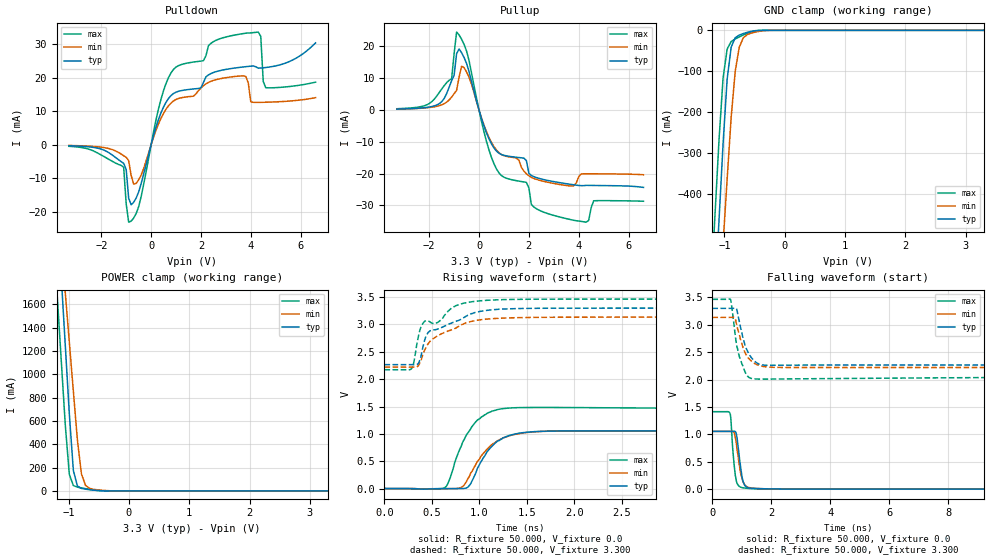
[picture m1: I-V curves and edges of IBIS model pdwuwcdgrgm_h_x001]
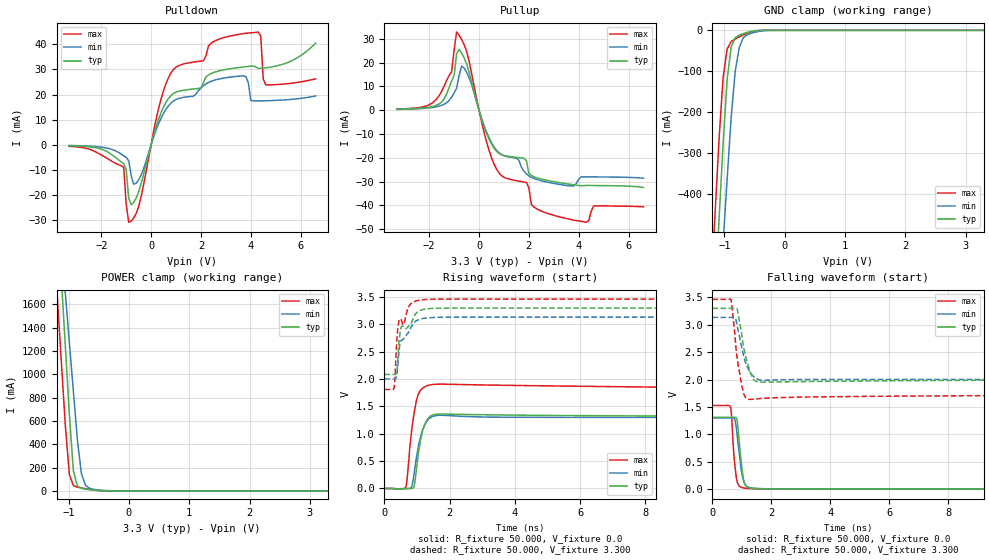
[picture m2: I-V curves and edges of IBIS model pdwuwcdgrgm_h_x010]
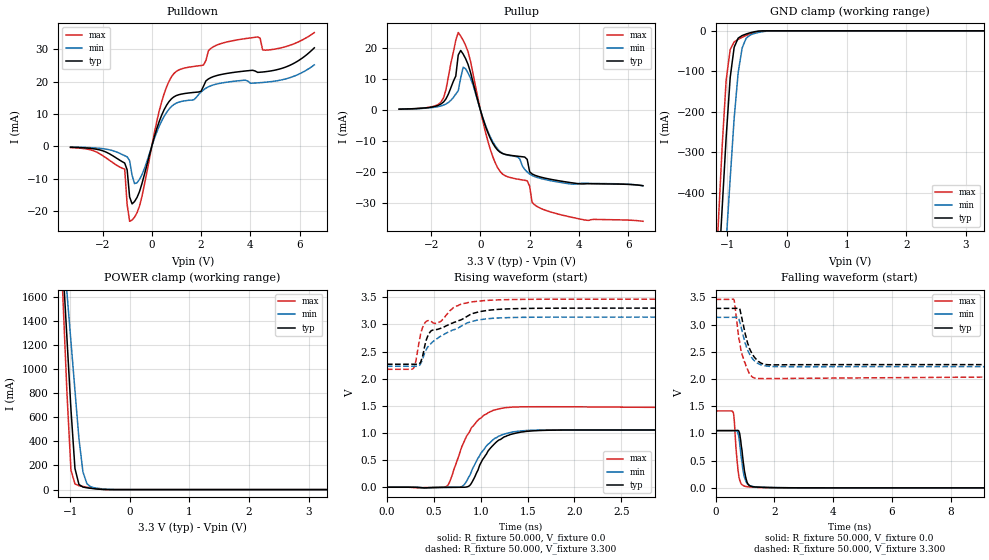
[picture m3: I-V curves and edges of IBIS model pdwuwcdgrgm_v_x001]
|   IBIS Model of Analog Devices ADSP-SC569
|   ADSP Device
[IBIS ver]   4.2
[File name]   adsc565.ibs
[File Rev]   1.0
[Date]   Fri Nov 29 10:39:13 IST 2019
[Source]   TSMC 28nm custom IO cells
[Notes]
|  GriffinUltraLite product standard
|This IBIS model is generated automatically using script /cad/local/apps/adi/ibis_gen/1.0/bin/chip_ibis_model_gen.pl
|No models exist for the following pins
|   ( Using type NC as a placeholder ):
|CLKIN_IN
|VIN0
|VIN1
|VIN2
|VIN3
|VREF_N_ADC
|VREF_P_ADC
[Disclaimer] Model intended for simulation purpose only.
[Copyright]   Property of Analog Devices Inc. Unauthorized reproduction and/or distribution is strictly prohibited.
[Component]   ADSP-SC569
[Manufacturer] Analog Devices Inc.
[Package]
|  variable   typ   min   max
R_pkg   339.97m   176.67m   530.1m
L_pkg   5.53nH   4.7nH   6.78nH
C_pkg   0.78pF   0.58pF   1.14pF
[Pin]   signal_name   model_name   R_pin   L_pin   C_pin
1	VDD_INT		POWER   NA	NA	NA
2	GND		GND   NA	NA	NA
3	VDD_INT		POWER   NA	NA	NA
4	VDD_INT		POWER   NA	NA	NA
5	CLKIN		NC   NA	NA	NA
6	XTAL		NC   NA	NA	NA
7	VDD_REF_EXT	POWER   NA	NA	NA
8	VDD_INT		POWER   NA	NA	NA
9	TEST		PDWUWCDGRGM_H			NA	NA	NA
10	CLKOUT		PDWUWCDGRGM_H			NA	NA	NA
11	VDD_REF_EXT	POWER   NA	NA	NA
12	VDD_EXT		POWER   NA	NA	NA
13	VDD_INT		POWER   NA	NA	NA
14	PA0		PDWUWCDGRGM_H			NA	NA	NA
15	PA1		PDWUWCDGRGM_H			NA	NA	NA
16	PA2		PDWUWCDGRGM_H			NA	NA	NA
17	VDD_INT		POWER   NA	NA	NA
18	PA3		PDWUWCDGRGM_H			NA	NA	NA
19	PA4		PDWUWCDGRGM_H			NA	NA	NA
20	PA5		PDWUWCDGRGM_H			NA	NA	NA
21	PA6		PDWUWCDGRGM_H			NA	NA	NA
22	VDD_INT		POWER   NA	NA	NA
23	VDD_REF_EXT	POWER   NA	NA	NA
24	VDD_EXT		POWER   NA	NA	NA
25	PA7		PDWUWCDGRGM_H			NA	NA	NA
26	PA8		PDWUWCDGRGM_H			NA	NA	NA
27	PA9		PDWUWCDGRGM_H			NA	NA	NA
28	PA10		PDWUWCDGRGM_H			NA	NA	NA
29	VDD_INT		POWER   NA	NA	NA
30	GND		GND   NA	NA	NA
31	GND		GND   NA	NA	NA
32	VDD_INT		POWER   NA	NA	NA
33	VDD_INT		POWER   NA	NA	NA
34	PA11		PDWUWCDGRGM_V			NA	NA	NA
35	PA12		PDWUWCDGRGM_V			NA	NA	NA
36	PA13		PDWUWCDGRGM_V			NA	NA	NA
37	PA14		PDWUWCDGRGM_V			NA	NA	NA
38	VDD_EXT		POWER   NA	NA	NA
39	VDD_REF_EXT	POWER   NA	NA	NA
40	PA15		PDWUWCDGRGM_V			NA	NA	NA
41	DAI0_P01	PDWUWCDGRGM_V			NA	NA	NA
42	DAI0_P02	PDWUWCDGRGM_V			NA	NA	NA
43	DAI0_P03	PDWUWCDGRGM_V			NA	NA	NA
44	VDD_INT		POWER   NA	NA	NA
45	VDD_INT		POWER   NA	NA	NA
46	DAI0_P04	PDWUWCDGRGM_V			NA	NA	NA
47	DAI0_P05	PDWUWCDGRGM_V			NA	NA	NA
48	DAI0_P06	PDWUWCDGRGM_V			NA	NA	NA
49	DAI0_P07	PDWUWCDGRGM_V			NA	NA	NA
50	VDD_EXT		POWER   NA	NA	NA
51	VDD_REF_EXT	POWER   NA	NA	NA
52	DAI0_P08	PDWUWCDGRGM_V			NA	NA	NA
53	DAI0_P09	PDWUWCDGRGM_V			NA	NA	NA
54	DAI0_P10	PDWUWCDGRGM_V			NA	NA	NA
55	DAI0_P19	PDWUWCDGRGM_V			NA	NA	NA
56	DAI0_P20	PDWUWCDGRGM_V			NA	NA	NA
57	VDD_INT		POWER   NA	NA	NA
58	GND		GND   NA	NA	NA
59	VDD_INT		POWER   NA	NA	NA
60	VDD_INT		POWER   NA	NA	NA
61	VDD_INT		POWER   NA	NA	NA
62	GND		GND   NA	NA	NA
63	DAI1_P20	PDWUWCDGRGM_H			NA	NA	NA
64	DAI1_P19	PDWUWCDGRGM_H			NA	NA	NA
65	DAI1_P10	PDWUWCDGRGM_H			NA	NA	NA
66	DAI1_P09	PDWUWCDGRGM_H			NA	NA	NA
67	VDD_REF_EXT	POWER   NA	NA	NA
68	VDD_EXT	POWER   NA	NA	NA
69	VDD_INT	POWER   NA	NA	NA
70	DAI1_P08	PDWUWCDGRGM_H			NA	NA	NA
71	DAI1_P07	PDWUWCDGRGM_H			NA	NA	NA
72	DAI1_P06	PDWUWCDGRGM_H			NA	NA	NA
73	DAI1_P05	PDWUWCDGRGM_H			NA	NA	NA
74	DAI1_P04	PDWUWCDGRGM_H			NA	NA	NA
75	DAI1_P03	PDWUWCDGRGM_H			NA	NA	NA
76	DAI1_P02	PDWUWCDGRGM_H			NA	NA	NA
77	DAI1_P01	PDWUWCDGRGM_H			NA	NA	NA
78	VDD_EXT		POWER   NA	NA	NA
79	VDD_REF_EXT	POWER   NA	NA	NA
80	VDD_INT		POWER   NA	NA	NA
81	VIN0		NC   NA	NA	NA
82	VIN1		NC   NA	NA	NA
83	VREF_P_ADC	NC   NA	NA	NA
84	VREF_N_ADC	NC   NA	NA	NA
85	VDD_A		POWER   NA	NA	NA
86	AGND		GND   NA	NA	NA
87	VDD_INT		POWER   NA	NA	NA
88	VDD_INT		POWER   NA	NA	NA
89	VDD_INT		POWER   NA	NA	NA
90	GND		GND   NA	NA	NA
91	VDD_INT		POWER   NA	NA	NA
92	GND		GND   NA	NA	NA
93	VDD_INT		POWER   NA	NA	NA
94	VDD_INT		POWER   NA	NA	NA
95	VDD_INT		POWER   NA	NA	NA
96	TDI		PDWUWCDGRGM_V			NA	NA	NA
97	TCK		PDWUWCDGRGM_V			NA	NA	NA
98	TMS		PDWUWCDGRGM_V			NA	NA	NA
99	TDO		PDWUWCDGRGM_V			NA	NA	NA
100	VDD_REF_EXT	POWER   NA	NA	NA
101	VDD_EXT		POWER   NA	NA	NA
102	FAULTb		PDWUWCDGRGM_V			NA	NA	NA
103	TRSTB		PDWUWCDGRGM_V			NA	NA	NA
104	RESETb		PDWUWCDGRGM_V			NA	NA	NA
105	BMODE0		PDWUWCDGRGM_V			NA	NA	NA
106	BMODE1		PDWUWCDGRGM_V			NA	NA	NA
107	RESOUTb		PDWUWCDGRGM_V			NA	NA	NA
108	PB0		PDWUWCDGRGM_V			NA	NA	NA
109	PB1		PDWUWCDGRGM_V			NA	NA	NA
110	VDD_INT		POWER   NA	NA	NA
111	VDD_EXT		POWER   NA	NA	NA
112	VDD_REF_EXT	POWER   NA	NA	NA
113	PB2		PDWUWCDGRGM_V			NA	NA	NA
114	PB3		PDWUWCDGRGM_V			NA	NA	NA
115	PB4		PDWUWCDGRGM_V			NA	NA	NA
116	PB5		PDWUWCDGRGM_V			NA	NA	NA
117	VDD_INT		POWER   NA	NA	NA
118	VDD_INT		POWER   NA	NA	NA
119	VDD_INT		POWER   NA	NA	NA
120	GND		GND   NA	NA	NA
|[Diff Pin] inv_pin   vdiff   tdelay_typ tdelay_min tdelay_max
[Model Selector] PDWUWCDGRGM_H
pdwuwcdgrgm_h_x001 Vbus 3.3V
pdwuwcdgrgm_h_x010 Vbus 3.3V
[Model Selector] PDWUWCDGRGM_V
pdwuwcdgrgm_v_x001 Vbus 3.3V
pdwuwcdgrgm_v_x010 Vbus 3.3V
| Models and submodels in the file (4): pdwuwcdgrgm_h_x001 (I/O), pdwuwcdgrgm_h_x010 (I/O), pdwuwcdgrgm_v_x001 (I/O), pdwuwcdgrgm_v_x010 (I/O)
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|   Model pdwuwcdgrgm_h
[Model] pdwuwcdgrgm_h_x001
Model_type I/O
Polarity   Non-Inverting
Enable   Active-Low
Vinl =  0.660V
Vinh =  2.640V
C_comp   1.489pF   1.448pF   1.508pF
C_comp_pullup   0.648pF   0.610pF   0.663pF
C_comp_pulldown   0.433pF   0.404pF   0.445pF
[Model Spec]
Vinh   2.640V   2.508V   2.772V
Vinl   0.660V   0.627V   0.693V
[Temperature Range]   25.000   0.125k   -40.000
[Voltage Range]   3.300V   3.135V   3.465V
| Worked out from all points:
|   slope of the pulldown table from 0 to 0.495 V, typ, clamps not added: 44.1 ohm
|   slope of the pullup table from 0 to 0.495 V, typ, clamps not added: 46.9 ohm
|   GND clamp passes 1 mA (typ) near -0.49 V on its own axis
|   POWER clamp passes 1 mA (typ) near -0.44 V on its own axis
|   rising waveform, R_fixture 50.000, V_fixture 0.0: 20-80 % time 232ps typ, 277ps min, 213ps max; typ from 0 V to 1.05 V
|   rising waveform, R_fixture 50.000, V_fixture 3.300: 20-80 % time 414ps typ, 371ps min, 331ps max; typ from 2.27 V to 3.3 V
|   falling waveform, R_fixture 50.000, V_fixture 0.0: 20-80 % time 151ps typ, 192ps min, 127ps max; typ from 1.05 V to 0 V
|   falling waveform, R_fixture 50.000, V_fixture 3.300: 20-80 % time 336ps typ, 361ps min, 222ps max; typ from 3.3 V to 2.27 V
[Pulldown]
|Voltage   I(typ)   I(min)   I(max)
-3.3V     -279uA     -202.5uA   -451.9uA
-1.1V     -5.541mA   -3.26mA    -6.734mA
-900mV    -15.94mA   -4.725mA   -23.11mA
-600mV    -15.91mA   -11.54mA   -20.53mA
400mV     9.624mA    7.961mA    13.71mA
1V        15.72mA    13.54mA    23.21mA
3.7V      23.25mA    20.61mA    33.22mA
4.3V      22.89mA    12.67mA    33.66mA
4.4V      22.93mA    12.68mA    32.39mA
4.5V      23mA       12.7mA     18.9mA
4.6V      23.08mA    12.71mA    17.05mA
6.6V      30.44mA    14.08mA    18.71mA
[Pullup]
|Voltage   I(typ)   I(min)   I(max)
-3.3V     304.3uA    281.9uA    413.9uA
-1.6V     1.978mA    1.36mA     5.473mA
-1.1V     9.211mA    4.075mA    9.817mA
-900mV    17.72mA    6.178mA    24.51mA
-600mV    16.54mA    13.33mA    20.64mA
600mV     -11.92mA   -11.52mA   -16.89mA
1.9V      -15.87mA   -20.02mA   -22.75mA
2.2V      -20.94mA   -21.51mA   -30.47mA
3.7V      -23.38mA   -23.88mA   -34.48mA
4.3V      -23.68mA   -20.04mA   -35.25mA
4.6V      -23.71mA   -20.04mA   -28.52mA
6.6V      -24.32mA   -20.34mA   -28.67mA
[GND_clamp]
|Voltage   I(typ)   I(min)   I(max)
-3.3V     -6.697A    -5.899A    -6.429A
-1.223V   -834.6mA   -989.4mA   -634mA
-1.156V   -647.4mA   -832.1mA   -449.2mA
-1.089V   -461.1mA   -675.2mA   -265.6mA
-1.022V   -276.3mA   -518.8mA   -115.9mA
-955mV    -119.5mA   -363.1mA   -45.68mA
-888mV    -40.94mA   -211.7mA   -27.28mA
-821mV    -18.09mA   -100.2mA   -21.05mA
-754mV    -11.69mA   -41.38mA   -15.99mA
-620mV    -4.821mA   -10.31mA   -7.225mA
-352mV    -29.83uA   -1.016mA   -30.26uA
3.3V      0A         0A         0A
[POWER_clamp]
|Voltage   I(typ)   I(min)   I(max)
-3.3V     21.13A     15.96A     19.27A
-1.189V   2.428A     2.545A     1.676A
-1.122V   1.837A     2.122A     1.121A
-1.055V   1.249A     1.699A     567.8mA
-988mV    663mA      1.276A     141.6mA
-921mV    174.9mA    855.3mA    46.28mA
-854mV    42.62mA    437.1mA    32.31mA
-787mV    21.33mA    146.3mA    25.61mA
-720mV    15.03mA    48.41mA    19.6mA
-653mV    10.52mA    22.14mA    14.03mA
-251mV    4.083uA    411.2uA    1.265uA
3.3V      0A         0A         0A
[Ramp]
| variable   typ   min   max
dV/dt_r   0.632/0.236n   0.632/0.277n   0.849/0.212n
dV/dt_f   0.621/0.334n   0.549/0.363n   0.779/0.229n
R_load = 50.000
[Rising Waveform]
R_fixture= 50.000
V_fixture= 0.0
V_fixture_min= 0.0
V_fixture_max= 0.0
|time   V(typ)   V(min)   V(max)
0s        334.6nV    124uV      235.4nV
640ps     -2.231mV   -1.827mV   21.16mV
690ps     -1.679mV   -1.21mV    184.2mV
800ps     -473uV     12.93mV    742mV
870ps     15.55mV    151.4mV    994.1mV
980ps     369.5mV    495.7mV    1.252V
1.08ns    669.5mV    715mV      1.374V
1.19ns    864.1mV    873.9mV    1.443V
1.47ns    1.024V     1.018V     1.482V
100ns     1.054V     1.054V     1.414V
[Rising Waveform]
R_fixture= 50.000
V_fixture= 3.300
V_fixture_min= 3.135
V_fixture_max= 3.465
|time   V(typ)   V(min)   V(max)
0s        2.265V     2.22V      2.173V
280ps     2.265V     2.22V      2.182V
310ps     2.265V     2.22V      2.31V
360ps     2.294V     2.253V     2.799V
410ps     2.618V     2.472V     3.031V
480ps     2.883V     2.692V     3.047V
750ps     3.056V     2.933V     3.343V
1ns       3.238V     3.083V     3.432V
1.53ns    3.295V     3.129V     3.462V
100ns     3.3V       3.135V     3.465V
[Falling Waveform]
R_fixture= 50.000
V_fixture= 0.0
V_fixture_min= 0.0
V_fixture_max= 0.0
|time   V(typ)   V(min)   V(max)
0s        1.054V     1.054V     1.414V
600ps     1.054V     1.054V     1.379V
630ps     1.054V     1.055V     1.268V
690ps     1.055V     1.055V     738.3mV
750ps     1.057V     1.013V     387mV
860ps     838.4mV    646.8mV    85.02mV
1ns       238.4mV    213.1mV    29.64mV
1.08ns    86.99mV    94.54mV    21.33mV
1.53ns    11.27mV    11.79mV    6.195mV
100ns     6.022uV    124.1uV    6.749uV
[Falling Waveform]
R_fixture= 50.000
V_fixture= 3.300
V_fixture_min= 3.135
V_fixture_max= 3.465
|time   V(typ)   V(min)   V(max)
0s        3.3V       3.135V     3.465V
620ps     3.3V       3.135V     3.459V
760ps     3.301V     3.13V      2.877V
820ps     3.292V     3.012V     2.643V
910ps     3.07V      2.831V     2.425V
1.13ns    2.591V     2.467V     2.116V
1.3ns     2.416V     2.349V     2.024V
1.51ns    2.304V     2.274V     2.01V
3.38ns    2.265V     2.22V      2.016V
100ns     2.265V     2.22V      2.167V
|   Model pdwuwcdgrgm_h
[Model] pdwuwcdgrgm_h_x010
Model_type I/O
Polarity   Non-Inverting
Enable   Active-Low
Vinl =  0.660V
Vinh =  2.640V
C_comp   1.490pF   1.443pF   1.504pF
C_comp_pullup   0.652pF   0.614pF   0.665pF
C_comp_pulldown   0.423pF   0.388pF   0.430pF
[Model Spec]
Vinh   2.640V   2.508V   2.772V
Vinl   0.660V   0.627V   0.693V
[Temperature Range]   25.000   0.125k   -40.000
[Voltage Range]   3.300V   3.135V   3.465V
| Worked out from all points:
|   slope of the pulldown table from 0 to 0.495 V, typ, clamps not added: 33.1 ohm
|   slope of the pullup table from 0 to 0.495 V, typ, clamps not added: 35.2 ohm
|   GND clamp passes 1 mA (typ) near -0.49 V on its own axis
|   POWER clamp passes 1 mA (typ) near -0.44 V on its own axis
|   rising waveform, R_fixture 50.000, V_fixture 0.0: 20-80 % time 204ps typ, 242ps min, 162ps max; typ from 0 V to 1.31 V
|   rising waveform, R_fixture 50.000, V_fixture 3.300: 20-80 % time 442ps typ, 386ps min, 316ps max; typ from 2.09 V to 3.3 V
|   falling waveform, R_fixture 50.000, V_fixture 0.0: 20-80 % time 153ps typ, 182ps min, 126ps max; typ from 1.31 V to 0 V
|   falling waveform, R_fixture 50.000, V_fixture 3.300: 20-80 % time 255ps typ, 318ps min, 215ps max; typ from 3.3 V to 2.08 V
[Pulldown]
|Voltage   I(typ)   I(min)   I(max)
-3.3V     -366.8uA   -266.9uA   -589.7uA
-1.1V     -7.472mA   -4.367mA   -8.993mA
-900mV    -21.24mA   -6.319mA   -30.8mA
-600mV    -21.2mA    -15.36mA   -27.35mA
400mV     12.82mA    10.6mA     18.26mA
1V        20.94mA    18.02mA    30.92mA
3.7V      30.97mA    27.44mA    44.25mA
4.3V      30.4mA     17.46mA    44.85mA
4.4V      30.46mA    17.48mA    43.24mA
4.5V      30.55mA    17.5mA     26.16mA
4.6V      30.66mA    17.52mA    23.89mA
6.6V      40.41mA    19.42mA    26.25mA
[Pullup]
|Voltage   I(typ)   I(min)   I(max)
-3.3V     406uA      356.1uA    503.1uA
-1.7V     2.105mA    1.472mA    4.778mA
-1.1V     12.29mA    5.477mA    16.17mA
-900mV    23.65mA    9.227mA    32.85mA
-600mV    22.06mA    17.82mA    27.59mA
600mV     -15.9mA    -15.37mA   -22.54mA
1.9V      -21.17mA   -26.69mA   -30.34mA
2.2V      -27.93mA   -28.67mA   -40.61mA
3.7V      -31.19mA   -31.85mA   -45.95mA
4.3V      -31.59mA   -28mA      -47.04mA
4.6V      -31.63mA   -28.01mA   -40.24mA
6.6V      -32.45mA   -28.56mA   -40.58mA
[GND_clamp]
|Voltage   I(typ)   I(min)   I(max)
-3.3V     -6.697A    -5.899A    -6.429A
-1.223V   -834.6mA   -989.4mA   -634mA
-1.156V   -647.4mA   -832.1mA   -449.2mA
-1.089V   -461.1mA   -675.2mA   -265.6mA
-1.022V   -276.3mA   -518.8mA   -115.9mA
-955mV    -119.5mA   -363.1mA   -45.68mA
-888mV    -40.94mA   -211.7mA   -27.28mA
-821mV    -18.09mA   -100.2mA   -21.05mA
-754mV    -11.69mA   -41.38mA   -15.99mA
-620mV    -4.821mA   -10.31mA   -7.225mA
-352mV    -29.83uA   -1.016mA   -30.26uA
3.3V      0A         0A         0A
[POWER_clamp]
|Voltage   I(typ)   I(min)   I(max)
-3.3V     21.13A     15.96A     19.27A
-1.189V   2.428A     2.545A     1.676A
-1.122V   1.837A     2.122A     1.121A
-1.055V   1.249A     1.699A     567.8mA
-988mV    663mA      1.276A     141.6mA
-921mV    174.9mA    855.3mA    46.28mA
-854mV    42.62mA    437.1mA    32.31mA
-787mV    21.33mA    146.3mA    25.61mA
-720mV    15.03mA    48.41mA    19.6mA
-653mV    10.52mA    22.14mA    14.03mA
-251mV    4.083uA    411.2uA    1.265uA
3.3V      0A         0A         0A
[Ramp]
| variable   typ   min   max
dV/dt_r   0.786/0.208n   0.780/0.246n   0.939/0.161n
dV/dt_f   0.730/0.256n   0.679/0.314n   1.004/0.214n
R_load = 50.000
[Rising Waveform]
R_fixture= 50.000
V_fixture= 0.0
V_fixture_min= 0.0
V_fixture_max= 0.0
|time   V(typ)   V(min)   V(max)
0s        279.1nV    104.9uV    196.5nV
650ps     -2.743mV   -2.307mV   17.96mV
690ps     -2.123mV   -1.782mV   148.2mV
840ps     61.07uV    44.38mV    1.09V
920ps     69.3mV     314.6mV    1.409V
990ps     398.5mV    603mV      1.631V
1.19ns    1.095V     1.096V     1.844V
1.36ns    1.298V     1.273V     1.89V
1.6ns     1.358V     1.336V     1.907V
100ns     1.311V     1.3V       1.566V
[Rising Waveform]
R_fixture= 50.000
V_fixture= 3.300
V_fixture_min= 3.135
V_fixture_max= 3.465
|time   V(typ)   V(min)   V(max)
0s        2.086V     2.003V     1.812V
290ps     2.086V     2.003V     1.833V
330ps     2.085V     2.004V     2.097V
380ps     2.159V     2.079V     2.702V
470ps     2.809V     2.615V     3.099V
590ps     2.961V     2.74V      3.003V
730ps     2.964V     2.851V     3.314V
920ps     3.162V     3.041V     3.418V
1.47ns    3.294V     3.127V     3.462V
100ns     3.3V       3.135V     3.465V
[Falling Waveform]
R_fixture= 50.000
V_fixture= 0.0
V_fixture_min= 0.0
V_fixture_max= 0.0
|time   V(typ)   V(min)   V(max)
0s        1.311V     1.3V       1.528V
620ps     1.311V     1.3V       1.491V
660ps     1.311V     1.3V       1.27V
740ps     1.312V     1.29V      550.8mV
820ps     1.293V     1.076V     189.6mV
860ps     1.172V     887.9mV    102.7mV
980ps     498.4mV    348.9mV    33.48mV
1.08ns    126.8mV    120.7mV    20.66mV
1.51ns    12.33mV    12.55mV    6.222mV
100ns     5.386uV    104.2uV    5.385uV
[Falling Waveform]
R_fixture= 50.000
V_fixture= 3.300
V_fixture_min= 3.135
V_fixture_max= 3.465
|time   V(typ)   V(min)   V(max)
0s        3.3V       3.135V     3.465V
630ps     3.3V       3.135V     3.459V
770ps     3.301V     3.132V     2.76V
840ps     3.289V     2.98V      2.394V
990ps     2.85V      2.609V     1.908V
1.09ns    2.521V     2.377V     1.701V
1.29ns    2.132V     2.129V     1.639V
1.44ns    1.981V     2.036V     1.643V
1.73ns    1.955V     1.988V     1.658V
100ns     2.083V     2.003V     1.792V
|   Model pdwuwcdgrgm_v
[Model] pdwuwcdgrgm_v_x001
Model_type I/O
Polarity   Non-Inverting
Enable   Active-Low
Vinl =  0.660V
Vinh =  2.640V
C_comp   1.509pF   1.450pF   1.564pF
C_comp_pullup   0.663pF   0.611pF   0.669pF
C_comp_pulldown   0.445pF   0.405pF   0.457pF
[Model Spec]
Vinh   2.640V   2.508V   2.772V
Vinl   0.660V   0.627V   0.693V
[Temperature Range]   25.000   0.125k   -40.000
[Voltage Range]   3.300V   3.135V   3.465V
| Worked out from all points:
|   slope of the pulldown table from 0 to 0.495 V, typ, clamps not added: 44.1 ohm
|   slope of the pullup table from 0 to 0.495 V, typ, clamps not added: 46.9 ohm
|   GND clamp passes 1 mA (typ) near -0.49 V on its own axis
|   POWER clamp passes 1 mA (typ) near -0.44 V on its own axis
|   rising waveform, R_fixture 50.000, V_fixture 0.0: 20-80 % time 232ps typ, 230ps min, 216ps max; typ from 0 V to 1.05 V
|   rising waveform, R_fixture 50.000, V_fixture 3.300: 20-80 % time 413ps typ, 388ps min, 331ps max; typ from 2.27 V to 3.3 V
|   falling waveform, R_fixture 50.000, V_fixture 0.0: 20-80 % time 158ps typ, 160ps min, 125ps max; typ from 1.05 V to 0 V
|   falling waveform, R_fixture 50.000, V_fixture 3.300: 20-80 % time 330ps typ, 342ps min, 229ps max; typ from 3.3 V to 2.27 V
[Pulldown]
|Voltage   I(typ)   I(min)   I(max)
-3.3V     -298.4uA   -220.2uA   -397.6uA
-1.1V     -5.197mA   -2.924mA   -7.067mA
-1V       -7.298mA   -3.281mA   -18.07mA
-900mV    -15.71mA   -4.45mA    -23.24mA
-600mV    -15.87mA   -11.3mA    -20.59mA
300mV     7.634mA    6.178mA    10.85mA
900mV     15.32mA    12.94mA    22.54mA
2.1V      18.6mA     17.46mA    25.13mA
2.9V      22.36mA    19.67mA    32.01mA
4.3V      22.89mA    19.64mA    33.86mA
4.8V      23.3mA     19.98mA    29.88mA
6.6V      30.48mA    25.21mA    35.22mA
[Pullup]
|Voltage   I(typ)   I(min)   I(max)
-3.3V     303.7uA    277uA      287.7uA
-1.6V     1.971mA    1.337mA    2.592mA
-1V       10.95mA    5.138mA    22.51mA
-900mV    17.74mA    6.202mA    24.95mA
-700mV    18.03mA    13.8mA     22.46mA
-600mV    16.54mA    13.27mA    20.81mA
300mV     -7.194mA   -6.78mA    -9.92mA
900mV     -14mA      -13.93mA   -20.61mA
1.9V      -15.87mA   -19.94mA   -22.76mA
2.1V      -20.57mA   -21.06mA   -29.71mA
2.7V      -22.04mA   -22.48mA   -32.41mA
6.6V      -24.34mA   -24.36mA   -35.8mA
[GND_clamp]
|Voltage   I(typ)   I(min)   I(max)
-3.3V     -6.331A    -5.928A    -6.883A
-1.156V   -612.4mA   -832mA     -480.5mA
-1.089V   -436.3mA   -675.2mA   -283.9mA
-1.022V   -261.8mA   -519.3mA   -121mA
-955mV    -115.5mA   -364.6mA   -46.32mA
-888mV    -40.48mA   -215.6mA   -27.35mA
-821mV    -18.03mA   -103.2mA   -21.08mA
-754mV    -11.67mA   -42.19mA   -16.02mA
-687mV    -7.883mA   -18.25mA   -11.37mA
-620mV    -4.816mA   -10.3mA    -7.232mA
-352mV    -29.83uA   -1.015mA   -30.22uA
3.3V      0A         0A         0A
[POWER_clamp]
|Voltage   I(typ)   I(min)   I(max)
-3.3V     21.2A      15.36A     27.27A
-1.189V   2.436A     2.445A     2.368A
-1.122V   1.844A     2.038A     1.583A
-1.055V   1.254A     1.632A     800mA
-988mV    665.4mA    1.226A     161.7mA
-921mV    175.4mA    823mA      47.01mA
-854mV    42.66mA    422.6mA    32.46mA
-787mV    21.34mA    146.7mA    25.7mA
-720mV    15.03mA    48.63mA    19.66mA
-653mV    10.52mA    22.18mA    14.07mA
-251mV    4.083uA    411.3uA    1.265uA
3.3V      0A         0A         0A
[Ramp]
| variable   typ   min   max
dV/dt_r   0.632/0.236n   0.630/0.229n   0.849/0.213n
dV/dt_f   0.620/0.334n   0.544/0.341n   0.779/0.228n
R_load = 50.000
[Rising Waveform]
R_fixture= 50.000
V_fixture= 0.0
V_fixture_min= 0.0
V_fixture_max= 0.0
|time   V(typ)   V(min)   V(max)
0s        335.1nV    125.7uV    199.3nV
630ps     -2.311mV   -2.183mV   11.96mV
670ps     -1.842mV   -1.641mV   105.3mV
820ps     -119.5uV   40.87mV    830.1mV
890ps     45.76mV    239.2mV    1.057V
980ps     362.4mV    556.3mV    1.252V
1.08ns    672.2mV    795.5mV    1.374V
1.19ns    865.4mV    939.3mV    1.441V
1.48ns    1.028V     1.044V     1.482V
100ns     1.054V     1.05V      1.415V
[Rising Waveform]
R_fixture= 50.000
V_fixture= 3.300
V_fixture_min= 3.135
V_fixture_max= 3.465
|time   V(typ)   V(min)   V(max)
0s        2.266V     2.228V     2.173V
280ps     2.266V     2.228V     2.185V
360ps     2.305V     2.278V     2.834V
400ps     2.579V     2.46V      3.015V
470ps     2.879V     2.647V     3.054V
570ps     2.925V     2.778V     3.052V
740ps     3.055V     2.921V     3.335V
1.01ns    3.241V     3.09V      3.433V
1.53ns    3.295V     3.131V     3.462V
100ns     3.3V       3.135V     3.465V
[Falling Waveform]
R_fixture= 50.000
V_fixture= 0.0
V_fixture_min= 0.0
V_fixture_max= 0.0
|time   V(typ)   V(min)   V(max)
0s        1.054V     1.05V      1.415V
610ps     1.054V     1.05V      1.371V
690ps     1.055V     1.05V      760.7mV
760ps     1.057V     1.011V     346.3mV
810ps     1.017V     863.3mV    167.5mV
860ps     846.2mV    623.2mV    83.47mV
970ps     361.3mV    220mV      35.79mV
1.08ns    93.2mV     73.66mV    21.55mV
1.53ns    11.26mV    12.26mV    6.21mV
100ns     6.316uV    125.3uV    7.396uV
[Falling Waveform]
R_fixture= 50.000
V_fixture= 3.300
V_fixture_min= 3.135
V_fixture_max= 3.465
|time   V(typ)   V(min)   V(max)
0s        3.3V       3.135V     3.465V
630ps     3.3V       3.135V     3.451V
780ps     3.302V     3.129V     2.801V
820ps     3.294V     3.052V     2.674V
870ps     3.177V     2.949V     2.513V
950ps     2.988V     2.776V     2.364V
1.15ns    2.566V     2.466V     2.1V
1.3ns     2.415V     2.347V     2.025V
1.55ns    2.292V     2.261V     2.009V
100ns     2.266V     2.228V     2.166V
